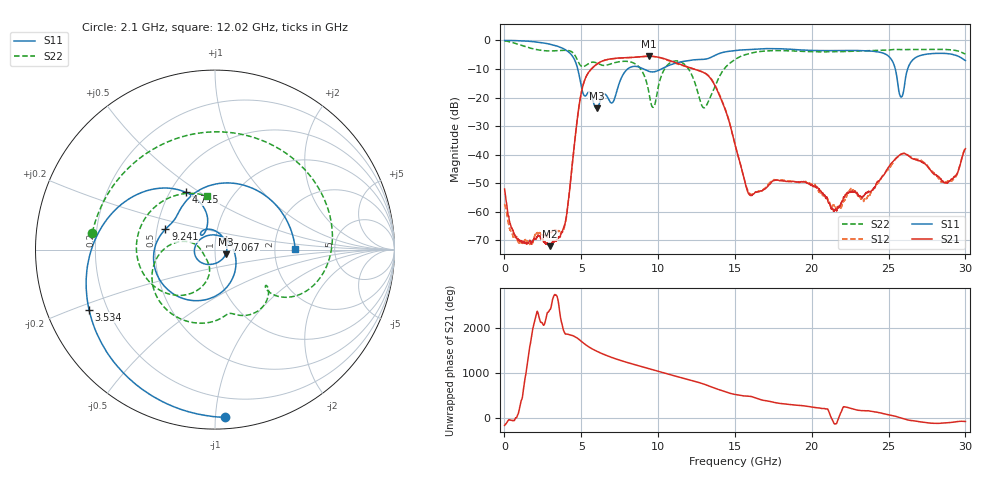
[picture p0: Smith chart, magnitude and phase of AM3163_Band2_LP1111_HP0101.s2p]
!Agilent Technologies,E8364B,MY43040894,A.07.50.67
!Agilent E8364B: A.07.50.67
!Date: Thursday, August 20, 2020 12:07:46
!Correction: S11(Full 2 Port(1,2))
!S21(Full 2 Port(1,2))
!S12(Full 2 Port(1,2))
!S22(Full 2 Port(1,2))
!S2P File: Measurements: S11, S21, S12, S22:
# Hz S  dB  R 50
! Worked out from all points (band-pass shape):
!   3201 points, 10 MHz to 30 GHz, reference 50 ohm
!   highest |S21| = -5.55 dB at 9.419 GHz (marker M1); lowest = -72.0 dB at 2.943 GHz (marker M2)
!   |S21| within 3 dB of the highest: 5.949 GHz to 11.53 GHz (5.58 GHz wide, 63.9 % of centre)
!   lowest |S11| = -23.8 dB at 5.999 GHz (marker M3), VSWR 1.14, Z = 56.2 - j2.94 ohm
!   |S11| at or under -10 dB: 4.77 GHz to 8.016 GHz (3.246 GHz wide, 50.8 % of centre); 9.056 GHz to 10.21 GHz (1.156 GHz wide, 12 % of centre); 25.44 GHz to 26.24 GHz (802.8 MHz wide, 3.11 % of centre)
!   |S22| runs from -23.6 to -0.2 dB; largest |S21 - S12| = 0.013
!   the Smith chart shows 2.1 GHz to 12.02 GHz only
!   S11 on the Smith chart (normalised r, x): 2.1 GHz: 0.07, -1.06; 3.534 GHz: 0.13, -0.22; 4.715 GHz: 0.60, +0.44; 7.067 GHz: 1.13, +0.13; 9.241 GHz: 0.55, +0.14; 12.02 GHz: 2.62, +0.02
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1e7  -0.01 -2.8  -51.97 -174.1  -57.19 174.4  -0.18 -7.0
9.190719e8  -0.10 -37.2  -69.89 111.8  -70.89 122.3  -1.39 -88.3
2.099928e9  -0.57 -86.6  -68.77 -159.5  -67.34 38.5  -3.22 172.1
2.943397e9  -1.30 -124.5  -72.01 -105.8  -67.20 -29.0  -3.68 106.5
3.533825e9  -2.18 -154.5  -68.88 1.9  -66.71 18.9  -3.56 61.8
4.714681e9  -8.94 116.9  -28.65 -12.7  -28.65 -13.2  -6.50 -34.2
5.014581e9  -16.54 106.3  -17.96 -93.4  -17.99 -93.7  -9.08 -36.8
5.998628e9  -23.77 -23.7  -8.34 49.4  -8.39 49.3  -7.90 -65.6
7.067022e9  -21.55 41.6  -6.35 -102.0  -6.41 -102.1  -7.95 -91.2
9.241297e9  -10.49 157.7  -5.57 33.0  -5.56 33.0  -14.49 166.0
9.419362e9  -10.86 151.0  -5.55 15.4  -5.53 15.3  -18.81 164.9
1.000979e10  -10.52 130.0  -5.86 -43.1  -5.90 -43.6  -16.28 -103.6
1.202474e10  -6.99 0.5  -9.47 129.2  -9.46 130.8  -10.38 99.0
1.301816e10  -6.59 -50.6  -11.38 26.7  -11.32 28.3  -23.57 -106.9
1.5005e10  -3.53 -132.6  -36.45 160.1  -36.41 159.4  -6.69 -112.3
1.597968e10  -3.19 -173.1  -54.11 119.1  -53.58 117.5  -4.54 -171.1
1.787279e10  -2.90 98.2  -49.02 -38.1  -48.95 -38.4  -3.57 91.9
2.000958e10  -3.50 -9.9  -50.75 -118.8  -50.33 -121.7  -3.93 -9.6
2.231506e10  -3.53 -100.0  -53.42 -130.7  -53.52 -140.1  -3.86 -93.8
2.500479e10  -5.54 157.7  -44.31 64.0  -45.07 67.6  -3.36 -167.8
2.582014e10  -19.81 171.2  -39.78 -7.7  -39.80 -8.2  -3.21 170.1
3e10  -7.04 50.8  -37.91 -86.1  -37.69 -86.0  -4.77 55.1
